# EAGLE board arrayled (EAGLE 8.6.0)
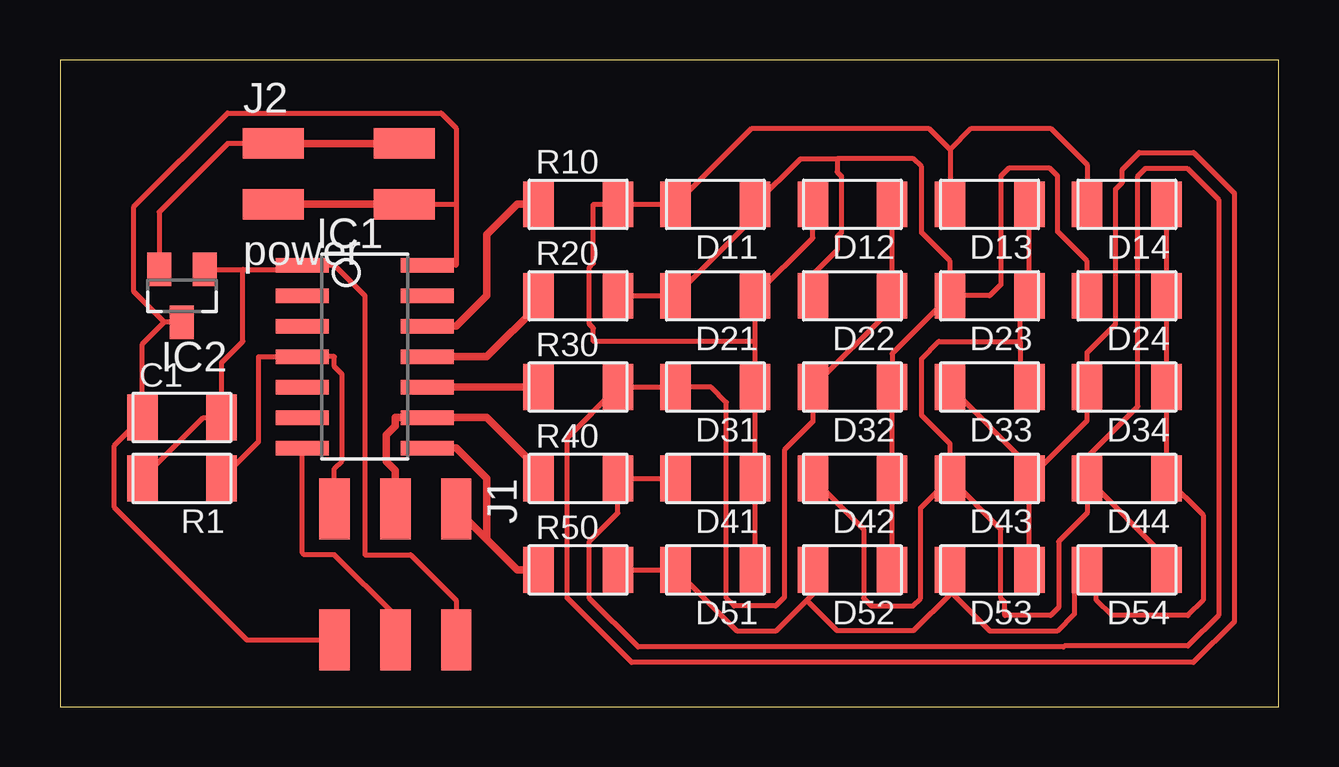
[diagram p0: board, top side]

Size 50.78 x 26.97 mm. Coordinates in mm from the lower left corner, seen from the top.
Outline: 0,0 50.78,0 50.78,26.97 0,26.97 0,0
Copper layers 1: Top 0.035mm
Design rules "basbasic": minimum track width 0.3mm, minimum drill 0.9mm, track to track 0.45mm, track to pad 0.45mm, pad to pad 0.45mm, via to via 0.45mm, smd to smd 6mil, copper to edge 40mil, drill to drill 6mil, minimum pad ring 10mil, minimum via ring 8mil, stop-mask expansion 4mil, vias tented up to drill 0mil, thermal gap 10mil

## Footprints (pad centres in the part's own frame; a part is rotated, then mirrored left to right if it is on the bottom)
C1206FAB = smd 1.27 x 1.905: 1 -1.651,0; 2 1.651,0
LED1206FAB = smd 1.27 x 1.905: 1 -1.651,0; 2 1.651,0
SOIC14 = smd 0.61 x 2.21: 1 -3.81,-2.603; 2 -2.54,-2.603; 3 -1.27,-2.603; 4 0,-2.603; 5 1.27,-2.603; 6 2.54,-2.603; 7 3.81,-2.603; 8 3.81,2.603; 9 2.54,2.603; 10 1.27,2.603; 11 0,2.603; 12 -1.27,2.603; 13 -2.54,2.603; 14 -3.81,2.603
SOT23 = smd 1 x 1.4: 1 -0.95,-1.1; 2 0.95,-1.1; 3 0,1.1
2X03SMD = smd 2.54 x 1.27: 1 -2.54,2.54; 2 2.92,2.54; 3 -2.54,0; 4 2.92,0; 5 -2.54,-2.54; 6 2.92,-2.54
2X02SMD = smd 2.54 x 1.27: 1 -2.54,1.27; 2 2.92,1.27; 3 -2.54,-1.27; 4 2.92,-1.27
R1206FAB = smd 1.27 x 1.905: 1 -1.651,0; 2 1.651,0

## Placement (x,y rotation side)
C1  1uF  [C1206FAB]  5.08,12.07 0 top
D11  LED  [LED1206FAB]  27.3,20.95 180 top
D12  LED  [LED1206FAB]  33.02,20.95 180 top
D13  LED  [LED1206FAB]  38.73,20.95 180 top
D14  LED  [LED1206FAB]  44.45,20.95 180 top
D21  LED  [LED1206FAB]  27.3,17.14 180 top
D22  LED  [LED1206FAB]  33.02,17.14 180 top
D23  LED  [LED1206FAB]  38.73,17.14 180 top
D24  LED  [LED1206FAB]  44.45,17.14 180 top
D31  LED  [LED1206FAB]  27.3,13.34 180 top
D32  LED  [LED1206FAB]  33.02,13.34 180 top
D33  LED  [LED1206FAB]  38.73,13.34 180 top
D34  LED  [LED1206FAB]  44.45,13.34 180 top
D41  LED  [LED1206FAB]  27.3,9.52 180 top
D42  LED  [LED1206FAB]  33.02,9.52 180 top
D43  LED  [LED1206FAB]  38.73,9.52 180 top
D44  LED  [LED1206FAB]  44.45,9.52 180 top
D51  LED  [LED1206FAB]  27.3,5.72 180 top
D52  LED  [LED1206FAB]  33.02,5.72 180 top
D53  LED  [LED1206FAB]  38.73,5.72 180 top
D54  LED  [LED1206FAB]  44.45,5.72 180 top
IC1  ATTINY44-SSU  [SOIC14]  12.7,14.61 270 top
IC2  5v  [SOT23]  5.08,17.14 180 top
J1  isp  [2X03SMD]  13.97,5.72 270 top
J2  power  [2X02SMD]  11.43,22.22 0 top
R1  10k  [R1206FAB]  5.08,9.52 180 top
R10  499  [R1206FAB]  21.59,20.95 0 top
R20  499  [R1206FAB]  21.59,17.14 0 top
R30  499  [R1206FAB]  21.59,13.34 0 top
R40  499  [R1206FAB]  21.59,9.52 0 top
R50  499  [R1206FAB]  21.59,5.72 0 top

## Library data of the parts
C1 D11-D14 D21-D24 D31-D34 D41-D44 D51-D54 IC1 IC2 J1 J2 R1 R10 R20 R30 R40 R50 = fab.lbr

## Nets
GND: C1.1 IC1.14 IC2.3 J1.6 J2.3 J2.4
MISO: IC1.8 J1.1 R50.1
MOSI: IC1.7 J1.4
RES1: IC1.12 R10.1
RES2: IC1.11 R20.1
RES3: IC1.10 R30.1
RESET: IC1.4 J1.5 R1.1
ROW1: D11.2 D12.2 D13.2 D14.2 D21.1 D31.1 D41.1 D51.1 R10.2
ROW2: D11.1 D21.2 D22.2 D23.2 D24.2 D32.1 D42.1 D52.1 R20.2
ROW3: D12.1 D22.1 D31.2 D32.2 D33.2 D34.2 D43.1 D53.1 R30.2
ROW4: D13.1 D23.1 D33.1 D41.2 D42.2 D43.2 D44.2 D54.1 R40.2
ROW5: D14.1 D24.1 D34.1 D44.1 D51.2 D52.2 D53.2 D54.2 R50.2
SCK: IC1.9 J1.3 R40.1
V+: IC2.2 J2.1 J2.2
VCC: C1.2 IC1.1 IC2.1 J1.2 R1.2

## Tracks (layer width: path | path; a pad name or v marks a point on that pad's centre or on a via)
GND
  Top 0.203: IC2.3 4.35,16.04 | 4.35,16.04 3.08,17.32 3.08,20.86 6.99,24.77 15.88,24.77 16.51,24.13 16.51,20.95 | 16.51,20.95 16.51,18.41 IC1.14 | J2.4 16.51,20.95 | J1.6 7.79,2.79 2.24,8.34 2.24,10.88 C1.1 3.43,15.12 4.35,16.04
  Top 0.305: J2.4 J2.3
MISO
  Top 0.305: IC1.8 16.51,10.8 17.78,9.52 17.78,6.99 | 17.78,6.99 19.05,5.72 R50.1 | J1.1 17.78,6.99
MOSI
  Top 0.203: J1.4 13.97,3.81 11.43,6.35 10.16,6.35 10.1,6.41 IC1.7
RES1
  Top 0.305: IC1.12 16.51,15.88 17.78,17.14 17.78,19.68 19.05,20.95 R10.1
RES2
  Top 0.305: IC1.11 17.78,14.61 19.94,16.76 R20.1
RES3
  Top 0.305: IC1.10 R30.1
RESET
  Top 0.203: R1.1 8.27,11.07 8.27,14.61 IC1.4 11.43,14.61 11.43,14.19 11.75,13.87 11.75,10.26 11.43,9.94 J1.5
ROW1
  Top 0.203: D12.2 31.37,19.56 D21.1 28.96,15.24 | 28.96,15.24 D31.1 D41.1 D51.1 | 28.96,15.24 22.23,15.24 22.23,15.79 22.05,15.96 22.05,18.33 22.23,18.5 22.23,20.95 R10.2 D11.2 28.83,24.13 36.2,24.13 37.08,23.24 | 37.08,23.24 D13.2 | 37.08,23.24 37.97,24.13 41.27,24.13 42.8,22.61 D14.2
ROW2
  Top 0.203: R20.2 D21.2 28.96,20.45 D11.1 30.86,22.86 32.38,22.86 | 32.38,22.86 32.38,22.31 32.56,22.14 32.56,19.77 32.38,19.6 32.38,19.05 31.37,18.03 D22.2 | D52.1 D42.1 D32.1 34.67,14.73 D23.2 | D24.2 42.8,18.59 41.57,19.81 41.57,22.14 41.25,22.46 39.52,22.46 39.2,22.14 39.2,17.61 38.73,17.14 D23.2 | D23.2 37.08,18.59 35.9,19.77 35.9,22.52 35.56,22.86 32.38,22.86
ROW3
  Top 0.203: D53.1 D43.1 | D12.1 D22.1 34.67,16.64 D32.2 31.37,11.89 30.18,10.71 30.18,4.57 29.82,4.21 28.09,4.21 27.77,4.53 27.77,12.7 27.13,13.34 D31.2 R30.2 21.13,11.22 21.13,4.54 23.81,1.85 47.22,1.85 48.93,3.56 48.93,21.42 47.23,23.11 44.97,23.11 44.26,22.41 44.26,21.87 43.99,21.59 43.99,15.96 42.8,14.78 D34.2 42.8,11.94 D43.1 | D33.2 40.39,10.03 D43.1
ROW4
  Top 0.203: D41.2 R40.2 23.24,8.08 22.05,6.9 22.05,4.53 24.09,2.5 41.82,2.5 41.85,2.54 46.99,2.54 48.28,3.83 48.28,21.14 46.96,22.46 45.24,22.46 44.91,22.14 44.91,12.53 42.8,10.41 D44.2 | D54.1 46.1,6.22 D44.2 | D44.2 42.8,8.08 41.61,6.9 41.61,4.15 41.27,3.81 39.37,3.81 39.37,4.36 39.2,4.53 39.2,7.41 D43.2 | 40.39,16.64 D23.1 | D23.1 D13.1 | D43.2 35.86,8.3 35.86,4.53 35.53,4.21 33.81,4.21 33.48,4.53 33.48,7.41 D42.2 | D43.2 37.08,10.97 35.9,12.15 35.9,14.52 36.62,15.24 40,15.24 | 40,15.24 40,13.72 D33.1 | 40,15.24 40,16.76 D23.1
ROW5
  Top 0.203: D14.1 D24.1 D34.1 D44.1 47.62,8 47.62,4.45 46.99,3.81 43.81,3.81 43.18,4.45 43.18,5.33 D54.2 42.27,5.18 42.27,3.88 41.55,3.16 38.75,3.16 37.08,4.83 D53.2 37.08,4.7 35.56,3.17 32.38,3.17 31.11,4.45 | R50.2 D51.2 28.19,3.17 29.84,3.17 31.11,4.45 | 31.11,4.45 31.37,4.7 D52.2
SCK
  Top 0.305: J1.3 13.97,9.87 13.6,10.24 13.6,11.35 13.97,11.72 13.97,12.07 IC1.9 17.78,12.07 19.94,9.91 R40.1
V+
  Top 0.203: J2.1 6.99,23.5 4.13,20.64 IC2.2
  Top 0.305: J2.2 J2.1
VCC
  Top 0.203: IC2.1 7.62,18.25 | 7.62,18.25 9.93,18.25 IC1.1 11.43,18.41 12.7,17.14 12.7,6.35 14.61,6.35 16.51,4.45 J1.2 | R1.2 5.97,12.07 C1.2 6.73,14.35 7.62,15.24 7.62,18.25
